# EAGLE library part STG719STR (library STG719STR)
STMICROELECTRONICS - STG719STR - IC, SWITCH, SPDT, SMD Source: Datasheet
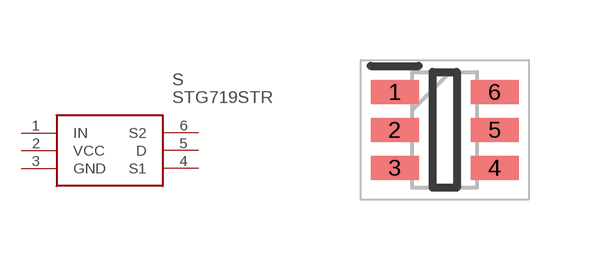
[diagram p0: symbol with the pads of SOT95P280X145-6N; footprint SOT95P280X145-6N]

Designator prefix S

## STG719STR (Arrow_Part_Number: STG719STR; Arrow_Price-Stock: https://www.arrow.com/en/products/stg719str/stmicroelectronics?region=nac; Description: STMICROELECTRONICS - STG719STR - IC, SWITCH, SPDT, SMD; Height: 1.45mm; Manufacturer_Name: STMicroelectronics; Manufacturer_Part_Number: STG719STR; Mouser_Part_Number: 511-STG719STR; Mouser_Price-Stock: https://www.mouser.co.uk/ProductDetail/STMicroelectronics/STG719STR?qs=tk5EcTX4n4wHN453KpBiVQ%3D%3D)  [SOT95P280X145-6N]
1  IN
2  VCC
3  GND
4  S1
5  D
6  S2

## Footprint SOT95P280X145-6N (pad centres in mm)
SOT23-6L_4
smd 1.2 x 0.6: 1 -1.25,0.95; 2 -1.25,0; 3 -1.25,-0.95; 4 1.25,-0.95; 5 1.25,0; 6 1.25,0.95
